(* Logix 5000 AddOnInstructionDefinition export AMCI_SD4840E2_Run_Dwell_Move; software revision 20.03 *)

ADD_ON_INSTRUCTION AMCI_SD4840E2_Run_Dwell_Move   (* revision 5.0, vendor AMCI, ExecuteEnableInFalse *)
// Revision note:
// Version 5.0 added the (hidden) ability to program the motor current and unlatched the error bit if the rung goes false.
VAR_INPUT
   Axis_Status_Bits : INT; {required}
   Type_0_for_standard_1_for_indexed : BOOL;
   motor_current : INT;
   Assembled_Move_Dwell_Time : INT; {required}
END_VAR
VAR_IN_OUT
   AMCI_SD4840E2_output_data : _000A:SD4840E2_4342D302:O:0; {required}
END_VAR
VAR_OUTPUT
   EN : BOOL; {visible}
   ER : BOOL; {visible}
END_VAR
VAR
   command_data_block : INT[10];
        [0]   // Command Bits MSW
        [1]   // Command Bits LSW
        [2]   // Upper Target Position
        [3]   // Lower Target Position
        [4]   // Upper Programmed Speed
        [5]   // Lower Programmed Speed
END_VAR

ROUTINE EnableInFalse   (* ladder *)
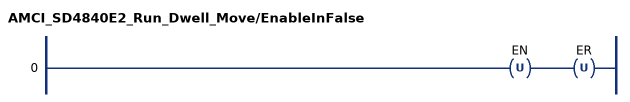
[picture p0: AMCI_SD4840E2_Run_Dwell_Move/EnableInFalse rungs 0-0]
   0: OTU(EN)OTU(ER);
END_ROUTINE

ROUTINE Logic   (* ladder *)
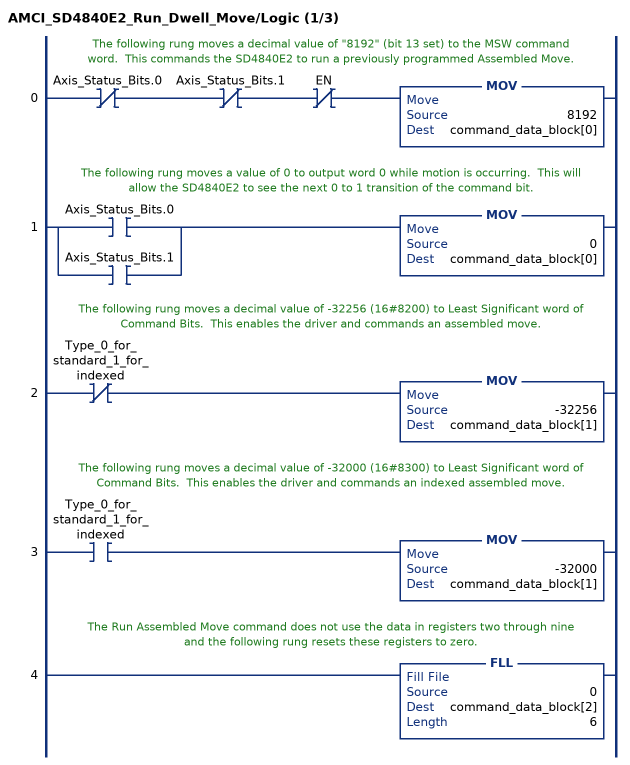
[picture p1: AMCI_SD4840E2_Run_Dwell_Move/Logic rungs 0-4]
   // The following rung moves a decimal value of "8192" (bit 13 set) to the MSW command word.  This commands the SD4840E2 to run a previously programmed Assembled Move.
   0: XIO(Axis_Status_Bits.0)XIO(Axis_Status_Bits.1)XIO(EN)MOV(8192,command_data_block[0]);
   // The following rung moves a value of 0 to output word 0 while motion is occurring.  This will allow the SD4840E2 to see the next 0 to 1 transition of the command bit.
   1: [XIC(Axis_Status_Bits.0) ,XIC(Axis_Status_Bits.1) ]MOV(0,command_data_block[0]);
   // The following rung moves a decimal value of -32256 (16#8200) to Least Significant word of Command Bits.  This enables the driver and commands an assembled move.
   2: XIO(Type_0_for_standard_1_for_indexed)MOV(-32256,command_data_block[1]);
   // The following rung moves a decimal value of -32000 (16#8300) to Least Significant word of Command Bits.  This enables the driver and commands an indexed assembled move.
   3: XIC(Type_0_for_standard_1_for_indexed)MOV(-32000,command_data_block[1]);
   // The Run Assembled Move command does not use the data in registers two through nine and the following rung resets these registers to zero.
   4: FLL(0,command_data_block[2],6);
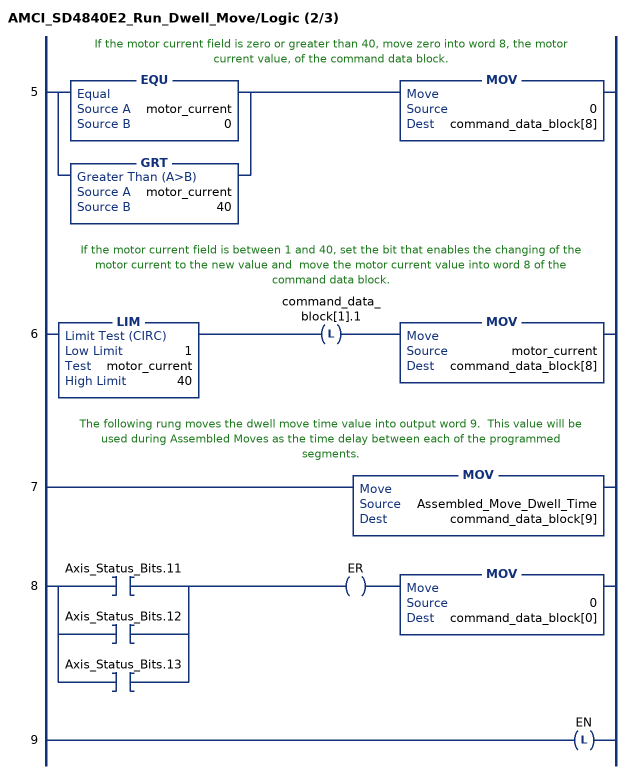
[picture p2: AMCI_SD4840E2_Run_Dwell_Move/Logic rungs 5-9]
   // If the motor current field is zero or greater than 40, move zero into word 8, the motor current value, of the command data block.
   5: [EQU(motor_current,0) ,GRT(motor_current,40) ]MOV(0,command_data_block[8]);
   // If the motor current field is between 1 and 40, set the bit that enables the changing of the motor current to the new value and  move the motor current value into word 8 of the command data block.
   6: LIM(1,motor_current,40)OTL(command_data_block[1].1)MOV(motor_current,command_data_block[8]);
   // The following rung moves the dwell move time value into output word 9.  This value will be used during Assembled Moves as the time delay between each of the programmed segments.
   7: MOV(Assembled_Move_Dwell_Time,command_data_block[9]);
   8: [XIC(Axis_Status_Bits.11) ,XIC(Axis_Status_Bits.12) ,XIC(Axis_Status_Bits.13) ]OTE(ER)MOV(0,command_data_block[0]);
   9: OTL(EN);
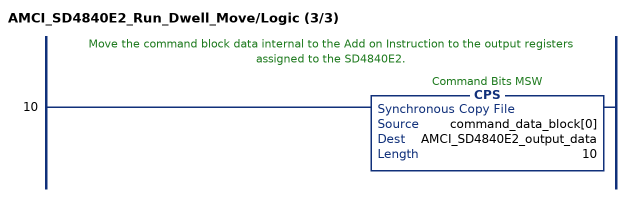
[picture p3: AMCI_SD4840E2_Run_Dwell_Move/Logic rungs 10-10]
   // Move the command block data internal to the Add on Instruction to the output registers assigned to the SD4840E2.
   10: CPS(command_data_block[0],AMCI_SD4840E2_output_data,10);
END_ROUTINE
END_ADD_ON_INSTRUCTION
